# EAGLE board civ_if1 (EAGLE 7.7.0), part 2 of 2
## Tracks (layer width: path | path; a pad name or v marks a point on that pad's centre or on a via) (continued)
N$93  (via drill 0.3) (continued)
  Bottom 0.254: v95.49,87.55 94.22,86.28 v94.22,85.88 | v93.9,79.77 v95.01,80.88 | v86.76,72.15 v88.19,73.58 | v75.41,71.68 v76.99,71.68 | v66.28,71.99 v67.31,73.03 | v64.21,71.83 63.9,71.83 62.55,70.48 62.07,70.48 v61.52,69.93
N$94  (via drill 0.3)
  Top 0.254: v127.24,71.91 130.89,71.91 136.53,77.55 136.53,83.34 137.4,84.22 137.4,86.04 139.38,88.03 142.16,88.03 143.27,89.14 143.27,97.23 142.88,97.63 141.05,97.63 140.49,97.08 140.49,93.74 140.1,93.34 138.03,93.34 137.24,94.14 135.49,94.14 135.25,94.38 130.81,94.38 R54.2 | v125.81,70.48 125.57,70.72 123.51,70.72 120.97,68.18 120.97,67.47 118.03,64.53 118.03,59.21 114.46,55.64 111.68,55.64 111.12,55.09 111.12,53.26 110.57,52.7 109.22,52.7 108.9,52.39 105.73,52.39 105.65,52.47 98.5,52.47 98.03,52.94 97.39,52.94 95.73,51.28 94.06,51.28 92.08,53.26 92.08,55.09 91.52,55.64 91.52,56.04 91.28,56.28 90.25,56.28 88.5,54.53 88.5,53.26 88.11,52.86 80.72,52.86 72.87,60.72 72.87,64.14 72.63,64.37 v72.63,64.69 | v71.2,63.26 71.44,63.02 71.44,60.4 65.56,54.53 v65.25,54.53 | v64.21,55.56 64.45,55.8 64.45,56.12 62.31,58.26 62.31,59.77 61.59,60.48 60.88,60.48 60.56,60.8 53.02,60.8 49.05,64.77 48.97,64.77 48.9,64.69 47.62,64.69 U1.11
  Bottom 0.254: v125.81,70.48 v127.24,71.91 | v71.2,63.26 v72.63,64.69 | v64.21,55.56 v65.25,54.53
N$95
  Top 0.61: D31.1 139.7,78.66 138.43,78.66 137.16,79.93 137.16,83.03 138.43,84.3 139.7,84.3 L1.2
N$96  (via drill 0.3)
  Top 0.254: v137.95,94.46 138.03,94.38 139.06,94.38 R55.2 | v136.92,93.42 136.92,87.95 136.45,87.47 135.41,87.47 126.13,78.18 118.51,78.18 116.36,76.04 114.62,76.04 113.98,76.68 v107.95,76.68 | v106.92,75.64 105.57,75.64 104.54,74.61 104.54,71.68 108.03,68.18 108.19,68.18 108.58,67.79 108.58,65.96 105.81,63.18 99.3,63.18 v99.06,63.42 | v97.63,62.07 97.63,62.39 85.72,74.3 v84.38,74.3 | v83.34,75.33 83.34,75.01 82.15,73.82 78.26,73.82 78.18,73.9 78.18,74.22 77.71,74.69 77.71,75.01 v76.99,75.72 | v75.41,75.72 67.71,75.72 v66.52,76.91 | v64.37,79.06 53.26,90.17 v51.28,90.17 | v50.24,89.14 50.48,88.9 50.48,82.87 47.78,80.17 47.15,80.17 46.99,80.01 46.99,79.14 46.75,78.9 46.75,78.66 45.64,77.55 v45.64,75.49 | v44.21,74.06 44.21,73.26 43.34,72.39 39.93,72.39 38.66,71.12 37.31,71.12 v37.07,71.36 | v36.04,70.33 36.35,70.33 36.51,70.17 37.86,70.17 44.05,63.98 46.2,63.98 46.28,63.9 47.62,63.9 U1.12
  Bottom 0.254: v136.92,93.42 v137.95,94.46 | v106.92,75.64 v107.95,76.68 | v99.06,63.42 97.71,62.07 v97.63,62.07 | v83.34,75.33 v84.38,74.3 | v75.41,75.72 v76.99,75.72 | v64.37,79.06 v66.52,76.91 | v50.24,89.14 v51.28,90.17 | v44.21,74.06 v45.64,75.49 | v36.04,70.33 v37.07,71.36
N$97  (via drill 0.3)
  Top 0.254: v137.64,92.71 137.79,92.87 140.34,92.87 140.97,93.5 140.97,94.38 141.6,94.38 R56.2 | v136.21,92.71 135.02,93.9 132.4,93.9 131.68,93.19 129.86,93.19 129.54,92.87 126.05,92.87 118.75,85.57 118.75,84.93 117.63,83.82 103.03,83.82 101.84,85.01 97.63,85.01 95.49,82.87 95.49,81.44 95.73,81.2 v95.73,80.17 | v94.61,79.06 90.96,79.06 88.58,76.68 88.58,76.44 88.82,76.2 88.82,75.41 89.06,75.17 89.06,72.39 98.74,62.71 107.95,62.71 108.27,63.02 109.38,63.02 110.65,64.29 111.28,64.29 111.68,63.9 111.68,63.26 111.28,62.87 110.65,62.87 109.86,62.07 108.74,62.07 108.43,61.75 105.65,61.75 103.58,59.69 103.58,55.8 103.5,55.72 102.39,55.72 102.23,55.88 101.92,55.88 101.76,56.04 101.44,56.04 101.28,55.88 100.97,55.88 98.74,53.66 v98.74,53.26 | v97.71,52.23 97.39,52.23 95.96,50.8 94.06,50.8 89.14,45.88 89.14,40.72 90.33,39.53 92.23,39.53 92.31,39.45 92.31,36.59 92.23,36.51 89.38,36.51 89.3,36.43 89.3,33.58 90.33,32.54 92.23,32.54 92.31,32.46 92.31,29.61 91.92,29.21 28.65,29.21 25.32,32.54 25.32,44.69 24.53,45.48 24.53,48.66 25.64,49.77 25.64,50.16 37.62,62.15 v39.13,62.15 | v40.16,63.18 42.47,63.18 42.78,63.5 45.96,63.5 46.35,63.1 47.62,63.1 U1.13
  Bottom 0.254: v136.21,92.71 v137.64,92.71 | v94.61,79.06 v95.73,80.17 | v97.71,52.23 v98.74,53.26 | v40.16,63.18 v39.13,62.15
N$98
  Top 0.254: D1.A 72.39,35 76.83,35 D2.A
N$99
  Top 0.254: R98.1 27.07,41.91 27.07,45.09 Q12.3 25.64,45.09 25,45.72 25,48.42 25.8,49.21 Q30.1
N$100
  Top 0.254: JP7.5 56.52,81.92 51.51,81.92 51.44,81.84 51.44,79.45 51.51,79.38 53.02,79.38 54.85,77.55 U1.57
N$101
  Top 0.254: JP7.1 52.7,80.41 55.64,77.47 U1.56
N$102
  Top 0.254: D3.A 72.39,41.99 76.83,41.99 D4.A
N$103
  Top 0.254: D5.A 90.81,35 95.25,35 D6.A
N$104
  Top 0.254: D7.A 90.81,41.99 95.25,41.99 D8.A
N$105
  Top 0.254: Q31.3 32.38,40.88 32.31,40.8 28.97,40.8 28.81,40.64 28.81,39.37 R97.1 28.81,39.29 28.81,38.1 28.89,38.02 29.69,38.02 30,37.7 32.15,37.7 32.23,37.78 33.42,37.78 Q32.1
N$106
  Top 0.254: 30.24,33.02 C145.2 | 30.24,33.02 29.84,33.42 28.57,33.42 R94.1 | ST2.2 30.16,30.8 30.16,32.94 30.24,33.02
N$107
  Top 0.254: Q24.3 101.6,53.58 102.23,52.94 105.89,52.94 105.97,52.86 108.66,52.86 108.82,53.02 108.82,54.13 108.9,54.21 109.86,54.21 OK2.2
N$108  (via drill 0.3)
  Top 0.254: LED8.1 141.84,124.38 135.33,124.38 134.14,125.57 129.06,125.57 128.75,125.25 127.08,125.25 126.92,125.09 126.76,125.09 126.05,124.38 124.86,124.38 LED7.1 124.78,124.38 117.16,124.38 116.36,125.17 112.16,125.17 112,125.02 111.92,125.02 111.76,125.17 109.93,125.17 109.14,124.38 107.95,124.38 LED6.1 107.79,124.38 106.6,124.38 103.19,127.79 100.33,127.79 99.69,127.16 v99.69,126.84 | v98.66,127.87 98.27,128.27 92.87,128.27 92.39,127.79 92.39,125.65 92.08,125.33 92.08,124.46 92,124.38 90.88,124.38 LED5.1 90.81,124.38 88.98,124.38 v88.66,124.7 | 73.1,124.38 73.82,124.38 LED4.1 73.98,124.38 75.09,124.38 75.17,124.46 75.17,126.52 75.64,127 78.03,127 78.5,126.52 80.01,126.52 v80.33,126.84 | 73.1,124.38 67.31,124.38 66.83,124.86 61.04,124.86 60.72,125.17 58.98,125.17 58.18,124.38 56.91,124.38 LED3.1 56.75,124.38 49.13,124.38 48.66,124.86 44.05,124.86 43.74,125.17 41.99,125.17 41.2,124.38 39.93,124.38 LED2.1 39.85,124.38 33.34,124.38 32.15,125.57 27.07,125.57 26.75,125.25 25,125.25 24.13,124.38 22.86,124.38 LED1.1 | JP9.1 70.48,118.27 v71.36,119.14 | v73.1,120.89 73.34,121.13 73.34,122.79 73.1,123.03 73.1,124.38 | v87.63,125.73 86.92,125.73 86.36,126.29 85.49,126.29 v84.85,126.92 | v81.36,127.87 v82.31,127.87
  Bottom 0.254: v99.69,126.84 v98.66,127.87 | v73.1,120.89 v71.36,119.14 | v87.63,125.73 v88.66,124.7 | v84.85,126.92 84.53,126.92 83.42,128.03 82.47,128.03 v82.31,127.87 | v80.33,126.84 v81.36,127.87
N$109  (via drill 0.3)
  Top 0.254: v27.23,124.54 27.07,124.38 25.88,124.38 LED1.3 | v28.26,123.51 28.26,123.83 28.73,124.3 31.99,124.3 32.86,123.43 37.86,123.43 38.42,122.87 54.69,122.87 55.17,122.4 65.25,122.4 65.96,121.68 69.14,121.68 v69.61,121.21 | v70.64,120.17 71.36,120.17 74.3,117.24 74.3,116.6 v74.61,116.28
  Bottom 0.254: v28.26,123.51 v27.23,124.54 | v70.64,120.17 v69.61,121.21 | v74.61,116.28 74.93,116.28 77.55,113.67 JP8.1
N$110  (via drill 0.3)
  Top 0.254: v39.93,127.08 38.73,127.08 36.51,124.86 33.58,124.86 32.38,126.05 25.88,126.05 LED1.4 | v41.2,127.87 42.07,128.75 68.9,128.75 v71.12,126.52 | v72.55,125.09 v72.15,125.49 | v73.82,123.35 73.82,119.86 75.25,118.43 75.56,118.43 76.04,117.95 78.34,117.95 v78.58,118.19
  Bottom 0.254: v39.93,127.08 40.4,127.08 v41.2,127.87 | v72.15,125.49 v71.12,126.52 | v72.55,125.09 72.55,124.62 v73.82,123.35 | v78.58,118.19 79.38,117.4 79.38,114.94 JP8.3
N$111  (via drill 0.3)
  Top 0.254: v70.8,122.79 68.74,122.79 68.58,122.63 66.44,122.63 65.72,123.35 55.64,123.35 55.17,123.83 48.97,123.83 48.42,124.38 42.86,124.38 LED2.3 | v71.99,123.67 71.99,121.28 72.07,121.21 72.07,120.89 75.01,117.95 75.33,117.95 75.72,117.55 75.72,116.92 75.33,116.52 v75.33,114.38 | v76.36,113.35 76.36,112.95 76.99,112.32 81.84,112.32 JP8.5
  Bottom 0.254: v70.8,122.79 71.12,122.79 v71.99,123.67 | v76.36,113.35 v75.33,114.38
N$112  (via drill 0.3)
  Top 0.254: v70.33,121.92 69.93,122.32 68.98,122.32 68.82,122.16 66.2,122.16 65.48,122.87 55.4,122.87 54.93,123.35 38.66,123.35 38.1,123.9 33.1,123.9 32.23,124.78 28.5,124.78 27.07,123.35 21.67,123.35 21.59,123.43 21.59,126.92 23.42,128.75 39.29,128.75 41.12,126.92 41.12,126.68 41.75,126.05 42.78,126.05 LED2.4 | v75.01,117.24 v71.36,120.89 | v76.04,116.2 76.04,116.52 76.83,117.32 76.83,117.4 76.91,117.47 84.38,117.47 84.45,117.4 v84.45,116.84
  Bottom 0.254: v71.36,120.89 v70.33,121.92 | v76.04,116.2 v75.01,117.24 | v84.45,116.84 84.45,114.94 JP8.7
N$113
  Top 0.254: JP8.9 87,114.94 76.91,114.94 74.3,112.32 68.26,112.32 68.02,112.55 68.02,118.59 71.52,122.08 71.52,123.11 70.72,123.9 67.07,123.9 66.6,124.38 59.93,124.38 LED3.3
N$114  (via drill 0.3)
  Top 0.254: v83.66,124.86 83.34,124.86 79.45,128.75 74.37,128.75 70.48,124.86 67.55,124.86 66.36,126.05 59.93,126.05 LED3.4 | v82.63,123.83 82.63,121.13 87,116.76 87,115.89 87.31,115.57 87.31,115.33 87.71,114.94 89.53,114.94 JP8.11
  Bottom 0.254: v82.63,123.83 v83.66,124.86
N$115  (via drill 0.3)
  Top 0.254: v79.38,124.38 76.91,124.38 LED4.3 | v80.41,123.35 80.8,122.95 80.8,120.97 v80.57,120.73 | v81.6,119.7 83.03,119.7 v83.19,119.54 | v84.61,120.97 86.2,120.97 86.28,121.05 86.92,121.05 87.55,120.41 92,120.41 92.08,120.33 92.08,115.33 92.55,114.86 92.55,114.46 JP8.13
  Bottom 0.254: v80.41,123.35 v79.38,124.38 | v81.6,119.7 v80.57,120.73 | v84.61,120.97 v83.19,119.54
N$116  (via drill 0.3)
  Top 0.254: v81.28,125.89 81.12,126.05 76.91,126.05 LED4.4 | v82.31,126.92 82.71,126.92 v83.11,127.32 | v84.14,126.29 84.45,126.29 84.53,126.21 84.85,126.21 85.25,125.81 86.12,125.81 v86.92,125.02 | v88.5,123.43 v87.95,123.98 | v89.93,121.13 v89.93,122 | v91.36,118.35 v90.49,119.22 | v93.27,118.35 93.66,118.35 94.61,117.4 94.61,114.94 JP8.15
  Bottom 0.254: v82.31,126.92 v81.28,125.89 | v84.14,126.29 v83.11,127.32 | v87.95,123.98 v86.92,125.02 | v89.93,122 v88.5,123.43 | v89.93,121.13 89.93,119.78 v90.49,119.22 | v93.27,118.35 v91.36,118.35
N$117  (via drill 0.3)
  Top 0.254: v97.31,122.63 97,122.63 95.25,124.38 93.9,124.38 LED5.3 | JP8.16 v95.89,121.21
  Bottom 0.254: v95.89,121.21 v97.31,122.63
N$118
  Top 0.254: JP8.14 92.55,117 92.55,120.57 92.39,120.73 92.39,122.79 92.55,122.95 92.55,125.09 92.87,125.41 92.87,126.05 93.82,126.05 LED5.4
N$119
  Top 0.254: JP8.12 91.6,115.41 91.6,115.09 92.08,114.62 92.08,112.47 92.23,112.32 97.79,112.32 102.47,117 102.47,117.08 103.11,117.71 103.74,117.71 103.98,117.47 110.81,117.47 110.89,117.55 110.89,122.87 112,123.98 112,124.3 111.92,124.38 110.89,124.38 LED6.3
N$120  (via drill 0.3)
  Top 0.254: v86.6,124.06 87,124.06 88.34,125.41 88.34,125.65 91.44,128.75 107.31,128.75 109.14,126.92 109.14,126.68 109.78,126.05 110.81,126.05 LED6.4 | v85.57,123.03 83.9,121.36 83.9,120.57 JP8.10
  Bottom 0.254: v85.57,123.03 v86.6,124.06
N$121  (via drill 0.3)
  Top 0.254: v103.43,117 111.05,117 111.36,117.32 111.36,122.63 113.43,124.7 116.13,124.7 116.92,123.9 123.11,123.9 123.67,123.35 126.05,123.35 126.21,123.51 126.21,123.83 126.76,124.38 127.79,124.38 LED7.3 | v102.39,118.03 102.16,118.27 100.65,118.27 96.2,122.71 94.14,122.71 93.9,122.95 93.27,122.95 92.87,122.56 92.87,121.6 v93.11,121.36 | v91.36,119.7 91.12,119.94 87.55,119.94 v86.6,118.98 | v85.17,117.55 85.17,116.76 JP8.8
  Bottom 0.254: v102.39,118.03 v103.43,117 | v93.11,121.36 91.44,119.7 v91.36,119.7 | v85.17,117.55 v86.6,118.98
N$122  (via drill 0.3)
  Top 0.254: v102.79,116.28 103.74,116.28 103.98,116.52 111.28,116.52 111.84,117.08 111.84,122.4 113.67,124.22 115.89,124.22 116.68,123.43 122.87,123.43 123.43,122.87 126.29,122.87 126.52,123.11 128.83,123.11 130.49,124.78 134.22,124.78 135.1,123.9 140.1,123.9 140.65,123.35 143.03,123.35 143.11,123.43 143.11,126.92 143.03,127 140.65,127 138.51,124.86 135.57,124.86 134.38,126.05 127.87,126.05 LED7.4 | v101.76,117.32 101.52,117.55 100.65,117.55 95.96,122.24 v93.58,122.24 | v91.68,122.24 91.04,122.87 89.69,122.87 89.06,122.24 88.5,122.24 v87.63,121.36 | v85.88,119.62 v86.6,120.33
  Bottom 0.254: v101.76,117.32 v102.79,116.28 | v91.68,122.24 v93.58,122.24 | v86.6,120.33 v87.63,121.36 | v85.88,119.62 85.88,119.3 83.19,116.6 JP8.6
N$123  (via drill 0.3)
  Top 0.254: v112.08,116.28 112.08,116.6 112.32,116.84 112.32,122.16 113.9,123.75 115.65,123.75 116.44,122.95 122.63,122.95 123.19,122.4 126.52,122.4 126.76,122.63 129.06,122.63 130.73,124.3 133.99,124.3 134.86,123.43 139.86,123.43 140.41,122.87 143.27,122.87 143.59,123.19 143.59,124.3 143.67,124.38 144.78,124.38 LED8.3 | v110.17,118.19 109.93,117.95 104.22,117.95 103.98,118.19 103.27,118.19 102.71,118.75 100.89,118.75 98.03,121.6 98.03,125.81 96.04,127.79 93.42,127.79 v93.11,127.48 | v91.68,127.48 91.2,127.48 v90.81,127.08 | v89.53,127.87 88.66,128.75 85.57,128.75 83.19,126.36 v83.19,126.05 | v81.28,124.14 81.28,120.41 80.8,119.94 v80.8,118.19
  Bottom 0.254: v110.17,118.19 v112.08,116.28 | v91.68,127.48 v93.11,127.48 | v90.81,127.08 90.33,127.08 v89.53,127.87 | v81.28,124.14 v83.19,126.05 | v80.8,118.19 80.8,116.36 JP8.4
N$124  (via drill 0.3)
  Top 0.254: v109.22,127.87 110.09,128.75 142,128.75 143.59,127.16 143.59,126.13 143.67,126.05 144.78,126.05 LED8.4 | v107.95,127.08 107.95,127.4 107.08,128.27 100.09,128.27 v98.35,126.52 | v97.31,125.49 95.33,125.49 v95.09,125.25 | v91.84,123.35 89.46,123.35 88.82,122.71 86.92,122.71 85.49,124.14 83.34,124.14 82.63,124.86 80.88,124.86 77.71,121.68 v77.71,118.67
  Bottom 0.254: v109.22,127.87 108.74,127.87 v107.95,127.08 | v97.31,125.49 v98.35,126.52 | v95.09,125.25 93.74,125.25 v91.84,123.35 | v77.71,118.67 77.71,116.6 JP8.2
PLUS-CIV  (via drill 0.3)
  Top 0.406: R27.2 101.84,42.55 101.84,40.01 R28.2 102,39.93 103.19,39.93 v103.27,39.85 | v106.44,30.48 105.25,29.29 104.3,29.29 104.22,29.37 102.79,29.37 102.71,29.29 101.76,29.29 99.77,31.27 99.77,36.2 99.85,36.27 100.01,36.27 100.09,36.35 100.09,37.47 R26.2 | v107.47,31.51 107.47,35.24 108.19,35.96 110.41,35.96 110.81,36.35 110.81,38.89 109.93,39.77 108.03,39.77 107.16,40.64 107.16,41.43 v106.05,42.55 106.12,42.7 105.89,42.94 104.78,42.94 R29.2 104.62,42.94 104.06,42.94 104.06,42.47 104.22,42.31 104.22,41.12 v104.38,40.96 | v103.27,54.77 103.5,55.01 104.78,55.01 R39.2 | C61.2 130.18,54.05 130.1,53.98 v129.22,53.98 | v82.23,53.98 82.15,54.05 82.15,55.24 R34.1 | v129.22,66.99 129.14,67.07 127.64,67.07 OK4.6 | v128.27,53.1 IC12.16
  Bottom 0.406: v129.22,66.99 v129.22,53.98 128.31,53.06 | 106.05,43.02 v106.05,42.55 | v82.23,53.98 82.87,54.61 103.19,54.61 | 103.19,54.61 103.82,53.98 v104.46,53.98 106.05,52.39 106.05,44.13 106.05,43.02 | 128.31,53.06 119.38,44.13 118.19,43.02 106.05,43.02 | v107.47,31.51 v106.44,30.48 | v103.27,54.77 103.19,54.61 | v104.38,40.96 v103.27,39.85 | v128.27,53.1 128.31,53.06
UART1
  Top 0.254: Q30.3 30.24,48.26 30.32,48.34 30.32,48.82 30.64,49.13 31.75,49.13 R99.1 31.83,49.13 33.02,49.13 33.73,49.85 33.73,50.09 34.37,50.72 41.83,50.72 44.69,53.58 49.05,53.58 50.16,54.69 50.16,56.44 50.01,56.59 50.01,59.05 U1.18
UART2
  Top 0.254: Q31.1 33.34,46.75 33.42,46.83 33.42,48.82 34.21,49.61 34.21,49.85 34.61,50.24 42.07,50.24 44.93,53.1 49.29,53.1 50.64,54.45 50.64,56.67 50.48,56.83 50.48,57.39 50.88,57.78 50.88,59.05 U1.19
UART3
  Top 0.254: Q2.3 39.13,48.26 39.21,48.34 39.21,48.82 39.53,49.13 40.64,49.13 R3.1 40.72,49.13 41.91,49.13 42.39,49.61 42.39,49.85 45.16,52.63 49.53,52.63 52.86,55.96 52.86,56.91 53.26,57.31 53.26,59.05 U1.22
UART4
  Top 0.254: Q3.1 42.23,46.75 42.31,46.83 42.31,48.82 43.1,49.61 43.1,49.85 45.4,52.15 49.77,52.15 53.34,55.72 53.34,56.67 53.74,57.07 53.74,57.47 54.05,57.78 U1.23
UART5
  Top 0.254: Q6.3 48.02,48.26 48.1,48.34 48.1,48.82 48.42,49.13 49.53,49.13 R8.1 49.61,49.13 50.64,49.13 50.72,49.21 50.72,50.72 50.88,50.88 50.88,51.83 52.15,53.1 57.23,53.1 58.02,53.9 58.02,59.05 U1.28
UART6
  Top 0.254: Q7.1 51.12,46.75 51.2,46.83 51.2,50.48 51.36,50.64 51.36,51.59 52.39,52.63 57.47,52.63 58.5,53.66 58.5,57.47 58.82,57.78 58.82,59.05 U1.29
UART7
  Top 0.254: Q10.3 56.91,48.26 56.99,48.34 56.99,48.82 57.31,49.13 58.42,49.13 R13.1 58.5,49.13 59.69,49.13 60.09,49.53 60.09,52.07 61.67,53.66 61.67,55.17 61.28,55.56 61.28,59.05 U1.32
UART8
  Top 0.254: Q11.1 60.01,46.75 60.09,46.83 60.09,48.82 60.56,49.29 60.56,51.83 63.02,54.29 63.98,54.29 64.93,55.24 64.93,56.36 62.79,58.5 62.79,60.01 62.23,60.56 62.23,60.64 62.87,60.64 U1.33
UART9
  Top 0.254: Q15.3 65.8,48.26 65.88,48.34 65.88,48.82 66.2,49.13 67.31,49.13 R18.1 67.39,49.13 68.58,49.13 71.68,52.23 71.68,57.47 71.91,57.71 71.91,63.66 70.48,65.09 65.72,65.09 65.33,64.69 62.87,64.69 U1.38
UART10  (via drill 0.3)
  Top 0.254: v67.15,54.37 66.83,54.37 65.88,53.42 65.88,51.28 63.5,48.9 63.5,48.58 63.34,48.42 63.34,48.1 63.5,47.94 63.5,47.62 63.9,47.23 65.56,47.23 65.8,46.99 65.8,46.91 66.52,46.2 66.91,46.2 67.39,45.72 68.5,45.72 68.9,45.32 Q16.1 | v65.8,55.8 66.12,55.8 67.71,57.39 67.71,63.34 66.67,64.37 v66.04,64.37 | v65.01,65.41 64.21,65.41 64.14,65.48 U1.39
  Bottom 0.254: v67.15,54.37 65.8,55.72 v65.8,55.8 | v65.01,65.41 v66.04,64.37
UART11
  Top 0.254: R23.1 86.36,49.13 85.09,49.13 84.22,48.26 Q19.3 82.15,48.26 82.07,48.34 82.07,50.16 81.99,50.24 81.28,50.24 78.74,52.78 78.74,53.42 75.96,56.2 72.55,56.2 72.15,56.59 72.15,57.23 72.39,57.47 72.39,63.9 70.72,65.56 68.02,65.56 66.12,67.47 64.61,67.47 64.21,67.87 U1.42
UART12  (via drill 0.3)
  Top 0.254: v88.82,52.55 88.82,51.36 89.77,50.4 89.77,49.77 89.61,49.61 89.61,48.74 87.87,46.99 87.87,46.83 87.31,46.28 Q20.1 | v87.79,53.58 88.03,53.82 88.03,56.83 v92.31,61.12 | v93.74,62.55 93.74,65.56 89.93,69.37 83.11,69.37 81.28,67.55 81.28,66.99 80.8,66.52 79.77,66.52 79.38,66.12 79.38,64.69 78.98,64.29 75.41,64.29 72.87,66.83 v72.87,67.15 | v71.83,66.12 71.83,66.44 71.6,66.67 67.63,66.67 66.36,67.94 64.85,67.94 64.14,68.66 62.87,68.66 U1.43
  Bottom 0.254: v87.79,53.58 v88.82,52.55 | v93.74,62.55 v92.31,61.12 | v71.83,66.12 v72.87,67.15
UART13  (via drill 0.3)
  Top 0.254: OK1.4 95.89,54.21 96.12,54.21 96.12,57.15 R31.1 96.12,57.23 96.12,58.42 92.71,61.83 91.52,61.83 v91.28,61.59 | v90.25,62.63 86.44,62.63 85.41,61.59 83.5,61.59 83.26,61.83 77.15,61.83 71.83,67.15 67.87,67.15 67.39,67.63 67.39,68.26 67.71,68.58 67.71,71.6 66.6,72.71 62.87,72.71 U1.48
  Bottom 0.254: v91.28,61.59 v90.25,62.63
UART14  (via drill 0.3)
  Top 0.254: v102.47,58.26 102.55,58.18 Q24.1 | v101.44,59.29 80.88,79.85 v76.99,79.85 | v75.49,81.36 70.8,81.36 68.9,79.45 67.31,79.45 62.39,74.53 61.28,74.53 61.28,74.3 U1.49
  Bottom 0.254: v101.44,59.29 v102.47,58.26 | v75.49,81.36 v76.99,79.85
UART15
  Top 0.254: R28.1 100.09,40.01 100.09,41.12 99.77,41.43 98.74,41.43 96.6,43.58 92,43.58 91.92,43.66 91.92,44.77 91.84,44.85 90.81,44.85 OK1.1
VCC  (via drill 0.3)
  Top 0.406: OSC1.4 OSC1.1 42.47,82.16 C54.1 41.83,82.23 v40.96,82.23 | v57.78,78.42 57.78,77.69 C12.1 58.04,77 U1.53 | U1.61 51.64,77.05 C37.1 51.12,77.57 v51.12,78.42 | U1.45 65.62,70.28 C38.1 66.46,71.12 v66.99,71.12 | U1.35 65.88,62.28 C11.1 66.46,62.87 v66.99,62.87 | U1.25 55.65,55.69 C36.1 56.52,54.83 v56.52,54.29 | U1.15 45.59,61.47 45.09,60.96 44.03,60.96 C13.1 43.71,60.64 v42.86,60.64 | v89.06,50.09 89.06,48.97 87.47,47.39 86.36,47.39 R23.2 | v90.09,51.12 90.09,54.21 90.81,54.21 OK1.6 90.96,54.21 91.52,54.21 91.52,54.85 v90.81,55.56 | C21.1 90.17,83.5 93.5,83.5 93.58,83.42 93.58,82.31 IC1.3 93.58,82.07 93.58,81.2 95.73,79.06 100.57,79.06 103.98,75.64 103.98,71.44 108.03,67.39 108.03,66.91 107.47,66.91 OK3.6 107.31,66.91 106.2,66.91 106.05,66.75 v106.05,66.67 | 81.04,38.1 81.04,39.37 R24.2 81.04,39.53 81.04,40.64 81.12,40.72 82.71,40.72 82.79,40.8 82.79,41.91 R22.2 | 81.04,38.1 81.04,36.83 R21.2 | R5.2 78.5,65.41 78.5,67.94 C19.1 76.2,67.94 | R19.2 62.63,39.37 62.63,36.83 R16.2 62.63,36.67 62.63,35.88 62.55,35.8 62.31,35.8 v62.25,35.87 | R14.2 53.74,39.37 53.74,36.83 R11.2 53.74,36.67 53.74,35.88 53.66,35.8 53.42,35.8 v53.36,35.87 | R9.2 44.85,39.37 44.85,36.83 R6.2 44.85,36.67 44.85,35.88 44.77,35.8 44.53,35.8 v44.47,35.87 | R4.2 35.96,39.37 35.96,36.83 R1.2 35.96,36.67 35.96,35.88 35.88,35.8 35.64,35.8 v35.58,35.87 | R96.2 27.07,36.83 27.07,39.37 R97.2 27.07,39.53 v27.07,40.48 | R98.2 28.81,41.91 28.81,41.35 29.37,41.35 29.84,41.83 v29.86,41.9 | R2.2 37.7,41.91 37.7,41.35 38.26,41.35 38.73,41.83 v38.76,41.9 | v32.7,47.31 32.62,47.39 31.75,47.39 R99.2
  Top 0.406: v46.83,43.02 46.67,43.02 46.59,42.94 46.59,41.91 R7.2 | v41.59,47.31 41.51,47.39 40.64,47.39 R3.2 | v55.48,43.02 55.48,41.91 R12.2 | v50.48,47.31 50.4,47.39 49.53,47.39 R8.2 | v64.37,43.02 64.37,41.91 R17.2 | v59.37,47.31 59.29,47.39 58.42,47.39 R13.2 | v68.26,47.31 68.18,47.39 67.31,47.39 R18.2 | v94.38,55.72 94.38,57.15 R31.2 | v114.62,52.31 114.78,52.47 116.2,52.47 R32.1 | C35.2 116.2,75.01 116.76,75.01 v117.16,74.61 | v130.33,74.69 131.44,74.69 R40.2 | v113.98,45.09 113.74,44.85 112.39,44.85 OK2.6 | v68.1,67.94 76.2,67.94 | v114.3,71.44 IC2.16 | v80.96,38.1 81.04,38.1 | v70.48,94.3 JP5.1 | v71.52,93.27 71.83,92.95 74.77,92.95 75.72,92 75.8,92 76.76,91.04 76.76,80.72 76.2,80.17 76.2,67.94
  Bottom 0.406: 42.86,48.58 v41.59,47.31 41.59,47.94 40.96,48.58 33.97,48.58 v32.7,47.31 32.7,44.74 | 42.86,48.58 46.99,48.58 | 46.99,48.58 49.53,48.58 50.48,47.62 v50.48,47.31 51.75,48.58 55.56,48.58 | 55.56,48.58 56.52,48.58 | 56.52,48.58 58.74,48.58 59.37,47.94 v59.37,47.31 60.64,48.58 64.45,48.58 | 64.45,48.58 67.63,48.58 | 67.63,48.58 68.26,47.94 v68.26,47.31 | v56.52,54.29 56.52,48.58 | v66.99,62.87 67.94,61.91 | 67.94,61.91 67.94,55.56 | 67.94,55.56 67.94,50.48 67.63,50.16 67.63,48.58 | v66.99,71.12 67.94,70.17 67.94,67.94 | 67.94,67.94 67.94,61.91 | 42.86,48.58 v42.86,60.64 40.96,62.55 40.96,78.42 | 40.96,78.42 v40.96,82.23 | 40.96,78.42 v51.12,78.42 51.12,79.38 | v53.02,84.45 52.7,84.14 JP7.2 51.12,81.6 51.12,79.38 | v57.78,78.42 56.83,79.38 51.12,79.38 | 32.7,44.74 v29.86,41.9 28.59,41.9 27.12,40.43 v27.07,40.48 | v35.58,35.87 38.76,39.04 v38.76,41.9 35.54,41.9 32.7,44.74 | v44.47,35.87 47.65,39.04 v47.65,41.9 46.99,42.55 46.99,43.02 | 46.99,43.02 46.99,48.58 | v53.36,35.87 56.53,39.04 v56.53,41.9 55.56,42.87 55.56,43.02 | 55.56,43.02 55.56,48.58 | v62.25,35.87 65.42,39.04 v65.42,41.9 64.45,42.87 64.45,43.02 | 64.45,43.02 64.45,48.58 | 75.56,55.56 v90.81,55.56 94.38,55.56 | 75.56,55.56 67.94,55.56 | v80.96,38.1 75.56,43.5 75.56,55.56 | v113.98,45.09 115.25,46.35 v115.25,51.44 114.5,52.19 | 114.5,52.19 106.05,60.64 | 106.05,60.64 v106.05,66.67 107.31,65.41 112.71,65.41 114.3,66.99 v114.3,71.44 114.3,74.3 114.62,74.61 v117.16,74.61 130.33,74.61 | 106.05,60.64 100.97,55.56 94.38,55.56 | v131.44,73.66 130.49,74.61 130.33,74.61 | v90.09,51.12 v89.06,50.09 | v46.83,43.02 46.99,43.02 | v55.48,43.02 55.56,43.02
  Bottom 0.406: v64.37,43.02 64.45,43.02 | v94.38,55.72 94.38,55.56 | v114.62,52.31 114.5,52.19 | v130.33,74.69 130.33,74.61 | v68.1,67.94 67.94,67.94 | v71.52,93.27 v70.48,94.3

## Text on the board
_tsilk: VCC | LEDs | VCC | LEDs | CIV-IF / V1.0 / DJ0ABR | +12 | GND | GND | GND | GND | GND | GND | GND | GND | GND | GND | CIV1 | CIV2 | CIV3 | CIV4 | CIV5 | CIV6 | CIV-EXT | EXT RS232 INT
